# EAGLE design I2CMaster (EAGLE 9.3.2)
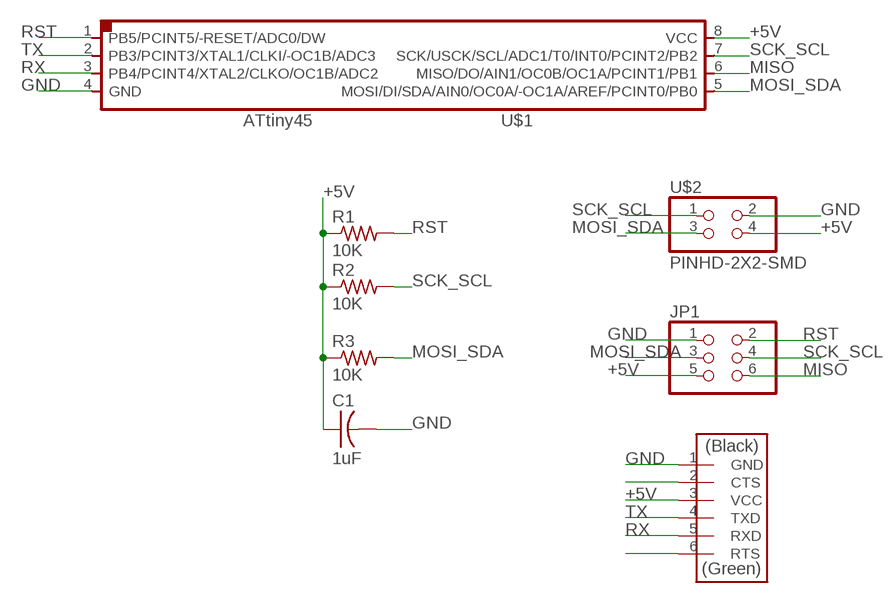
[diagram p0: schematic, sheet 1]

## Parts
C1  1uF  CAP-US1206FAB  [C1206FAB]
JP1  PINHD-2X3-SMD  [2X03SMD]
R1  10K  RES-US1206FAB  [R1206FAB]
R2  10K  RES-US1206FAB  [R1206FAB]
R3  10K  RES-US1206FAB  [R1206FAB]
U$1  ATTINY45SI  [SOIC8]
U$2  PINHD-2X2-SMD  [2X02SMD]
U$3  FTDI-SMD-HEADER  [1X06SMD]

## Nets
+5V: C1.1 JP1.5 R1.1 R2.1 R3.1 U$1.8(VCC) U$2.4 U$3.3(VCC)
GND: C1.2 JP1.1 U$1.4(GND) U$2.2 U$3.1(GND)
MISO: JP1.6 U$1.6(MISO/DO/AIN1/OC0B/OC1A/PCINT1/PB1)
MOSI_SDA: JP1.3 R3.2 U$1.5(MOSI/DI/SDA/AIN0/OC0A/-OC1A/AREF/PCINT0/PB0) U$2.3
N$2: U$3.2(CTS)
N$6: U$3.6(RTS)
RST: JP1.2 R1.2 U$1.1(PB5/PCINT5/-RESET/ADC0/DW)
RX: U$1.3(PB4/PCINT4/XTAL2/CLKO/OC1B/ADC2) U$3.5(RXD)
SCK_SCL: JP1.4 R2.2 U$1.7(SCK/USCK/SCL/ADC1/T0/INT0/PCINT2/PB2) U$2.1
TX: U$1.2(PB3/PCINT3/XTAL1/CLKI/-OC1B/ADC3) U$3.4(TXD)

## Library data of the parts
C1 = fab:CAP-US
JP1 = fab:PINHD-2X3-SMD: PIN HEADER
R1-R3 = fab:RES-US: Resistor (US Symbol)
U$1 = fab:ATTINY45
U$2 = fab:PINHD-2X2-SMD
U$3 = fab:FTDI-SMD-HEADER

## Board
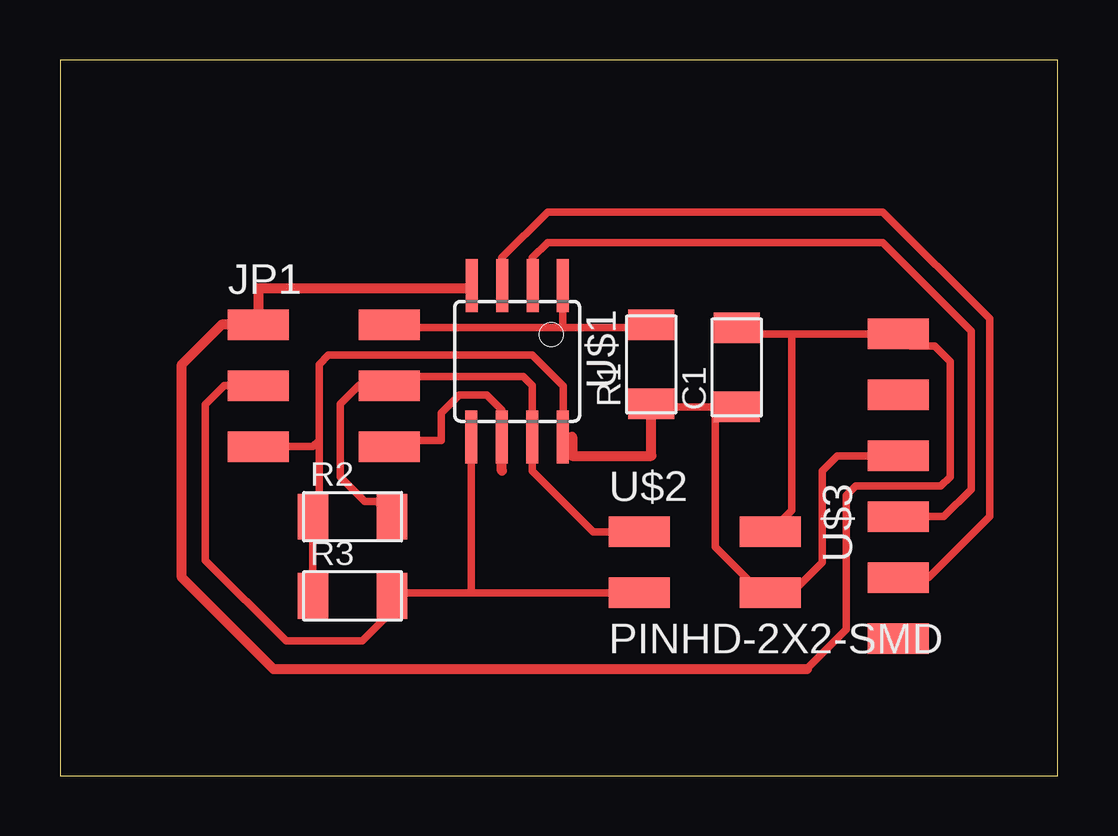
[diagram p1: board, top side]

Size 41.58 x 29.84 mm. Coordinates in mm from the lower left corner, seen from the top.
Outline: 0,0 41.58,0 41.58,29.84 0,29.84 0,0
Copper layers (1*16): Top 0.035mm / dielectric 1.5mm / Bottom 0.035mm
Design rules "default *": minimum track width 6mil, minimum drill 0.35mm, track to track 0.45mm, track to pad 0.45mm, pad to pad 0.45mm, via to via 0.45mm, smd to smd 0.45mm, copper to edge 0.4mm, drill to drill 0.4mm, minimum pad ring 10mil, minimum via ring 8mil, stop-mask expansion 4mil, vias tented up to drill 0mil, thermal gap 10mil

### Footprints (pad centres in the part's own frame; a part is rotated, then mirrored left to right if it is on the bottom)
C1206FAB = smd 1.27 x 1.905: 1 -1.651,0; 2 1.651,0
2X03SMD = smd 2.54 x 1.27: 1 -2.54,2.54; 2 2.92,2.54; 3 -2.54,0; 4 2.92,0; 5 -2.54,-2.54; 6 2.92,-2.54
R1206FAB = smd 1.27 x 1.905: 1 -1.651,0; 2 1.651,0
SOIC8 = smd 0.5 x 2.2: 1 -1.905,-3.154; 2 -0.645,-3.154; 3 0.625,-3.154; 4 1.895,-3.154; 5 1.905,3.154; 6 0.635,3.154; 7 -0.635,3.154; 8 -1.905,3.154
2X02SMD = smd 2.54 x 1.27: 1 -2.54,1.27; 2 2.92,1.27; 3 -2.54,-1.27; 4 2.92,-1.27
1X06SMD = smd 2.54 x 1.27: 1 0,6.35; 2 0,3.81; 3 0,1.27; 4 0,-1.27; 5 0,-3.81; 6 0,-6.35

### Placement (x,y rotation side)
C1  28.19,17.02 90 top
JP1  10.79,16.26 0 top
R1  24.64,17.14 90 top
R2  12.19,10.79 0 top
R3  12.19,7.49 0 top
U$1  19.05,17.27 180 top
U$2  26.67,8.89 0 top
U$3  34.92,12.06 0 top

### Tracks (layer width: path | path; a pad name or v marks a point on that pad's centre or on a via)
+5V
  Top 0.305: C1.1 27.3,15.37 | 27.3,15.37 24.77,15.37 R1.1 | 27.3,15.37 27.3,9.53 29.21,7.62 U$2.4 30.48,7.62 31.75,8.89 31.75,12.7 32.38,13.34 U$3.3 | 20.98,14.1 U$1.8 | 10.79,13.97 10.79,17.14 11.18,17.53 19.68,17.53 20.98,16.23 20.98,14.1 | 20.98,14.1 20.98,13.97 | JP1.5 10.54,13.72 10.79,13.97 | 10.79,13.97 10.79,11.05 R2.1 R3.1
  Top 0.406: 20.98,13.97 20.98,14.12 U$1.8 21.34,14.12 21.34,13.34 24.64,13.34 R1.1
GND
  Top 0.305: U$2.2 30.48,11.05 30.48,18.41 | 30.48,18.41 28.45,18.41 C1.2 | 30.48,18.41 U$3.1 35.43,17.91 36.45,17.91 37.08,17.27 37.08,12.45 36.7,12.06 33.15,12.06 32.77,11.68 32.77,6.1 31.11,4.45
  Top 0.406: 31.11,4.45 8.89,4.45 5.08,8.26 5.08,17.14 6.73,18.8 JP1.1 8.26,20.32 17.05,20.32 U$1.4
MISO
  Top 0.305: JP1.6 13.97,13.97 15.88,13.97 15.88,15.11 16.64,15.88 17.78,15.88 18.41,15.24 U$1.6
  Top 0.406: 18.41,12.7 U$1.6
MOSI_SDA
  Top 0.305: 17.14,7.62 13.97,7.62 R3.2 13.84,6.86 12.59,5.61 9.42,5.61 6.05,8.98 6.05,15.47 6.84,16.26 JP1.3 | 17.14,7.62 U$2.3 | U$1.5 17.14,7.62
RST
  Top 0.305: R1.2 24.51,18.8 24.38,18.67 20.95,18.67 | U$1.1 20.95,18.67 | 20.95,18.67 13.84,18.67 JP1.2
RX
  Top 0.305: U$3.5 36.2,8.26 38.73,10.79 38.73,19.05 34.29,23.5 20.32,23.5 18.41,21.59 18.43,21.58 U$1.3
SCK_SCL
  Top 0.305: U$2.1 22.23,10.16 19.68,12.7 U$1.7 19.68,16.26 19.3,16.64 14.1,16.64 JP1.4 12.45,16.26 11.68,15.49 11.68,12.45 12.7,11.43 13.21,11.43 R2.2
TX
  Top 0.305: U$3.4 36.83,10.79 37.97,11.94 37.97,18.54 34.29,22.23 20.32,22.23 19.68,21.59 19.68,20.44 U$1.2

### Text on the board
Reference: GND | GND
